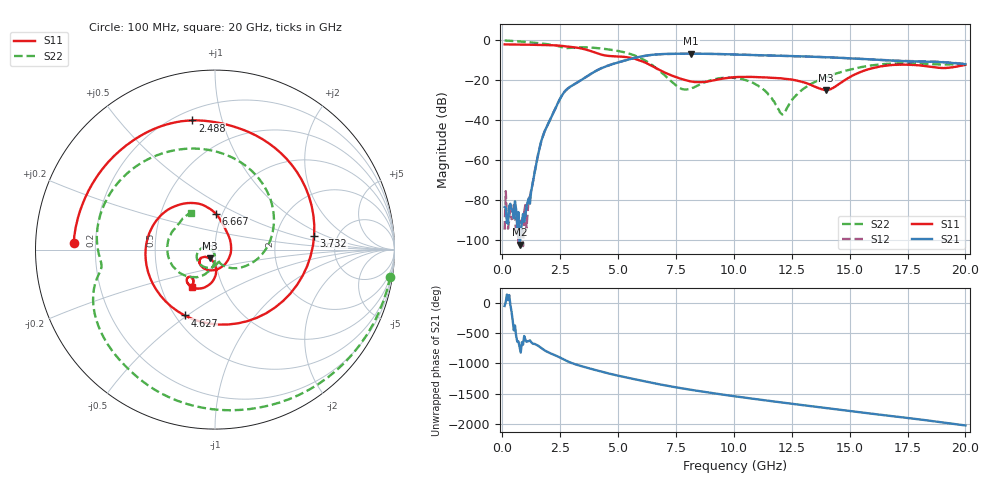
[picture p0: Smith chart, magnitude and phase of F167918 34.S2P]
!  2-Port S-parameters saved by WinCal
! VAR MeasName=S-Parameters (CALIBRATED_DATA) read from VNA (N5242A)
! VAR MeasDate=2016-11-22 10:26:23
! VAR NAME=F167918 34
! VAR FILENAME=F167918 34.S2P
! VAR DATE=2016-11-22 10:26:23
! VAR PHYS_PORTS=1,2
# Hz S DB R 50
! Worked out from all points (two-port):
!   401 points, 100 MHz to 20 GHz, reference 50 ohm
!   highest |S21| = -6.71 dB at 8.159 GHz (marker M1); lowest = -102.2 dB at 746.8 MHz (marker M2)
!   |S21| within 3 dB of the highest: 5.425 GHz to 16.13 GHz (10.71 GHz wide, 99.3 % of centre)
!   lowest |S11| = -25.0 dB at 13.98 GHz (marker M3), VSWR 1.12, Z = 47 - j4.57 ohm
!   |S11| at or under -10 dB: 5.912 GHz to end of sweep
!   |S22| runs from -37.2 to -0.1 dB; largest |S21 - S12| = 0.005
!   S11 on the Smith chart (normalised r, x): 100 MHz: 0.12, +0.02; 2.488 GHz: 0.26, +0.81; 3.732 GHz: 3.33, +0.76; 4.627 GHz: 0.56, -0.49; 6.667 GHz: 0.94, +0.39; 20 GHz: 0.71, -0.31
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1e8  -2.07 177.3  -83.38 -55.3  -94.75 -139.9  -0.10 -8.8
7.4675e8  -2.16 160.0  -102.19 -10.8  -90.54 164.3  -0.58 -59.8
1.14475e9  -2.23 149.0  -79.05 85.4  -79.16 60.4  -0.97 -87.8
1.74175e9  -2.35 130.4  -48.39 -44.1  -48.23 -44.0  -1.68 -124.7
2.488e9  -2.72 100.0  -29.37 176.0  -29.40 175.8  -3.19 -164.3
3.43325e9  -4.15 39.0  -19.71 31.1  -19.73 31.2  -3.51 163.5
3.73175e9  -5.07 8.1  -17.48 -0.6  -17.49 -0.4  -3.60 149.8
4.22925e9  -7.02 -58.5  -14.26 -52.3  -14.22 -52.1  -4.07 126.3
4.62725e9  -7.87 -114.8  -12.45 -90.8  -12.39 -91.0  -4.64 106.7
5.7715e9  -9.47 136.1  -8.65 172.7  -8.68 172.3  -7.87 38.1
6.667e9  -14.09 87.9  -7.06 102.2  -7.10 102.1  -14.12 -27.1
6.7665e9  -14.69 84.3  -6.98 94.8  -7.02 94.7  -15.05 -34.2
8.1595e9  -20.62 17.4  -6.71 2.4  -6.73 2.3  -24.12 -71.3
1.005e10  -18.44 -105.3  -7.11 -104.6  -7.12 -104.5  -18.85 -149.4
1.1244e10  -18.51 -133.2  -7.52 -165.5  -7.50 -165.5  -24.23 167.9
1.208975e10  -19.13 -141.8  -7.79 153.0  -7.76 152.9  -37.15 -141.1
1.338325e10  -22.70 -146.2  -8.22 90.3  -8.21 90.4  -21.57 -95.1
1.398025e10  -24.96 -120.8  -8.50 61.9  -8.47 61.8  -18.50 -104.1
1.527375e10  -16.89 -88.9  -9.20 0.8  -9.16 0.6  -13.99 -130.1
1.67165e10  -12.53 -113.5  -10.05 -65.8  -10.04 -65.8  -11.76 -165.4
1.865675e10  -13.50 -133.9  -10.75 -156.6  -10.70 -156.8  -12.02 150.2
2e10  -12.22 -122.3  -11.92 135.3  -11.83 135.1  -12.23 123.0
